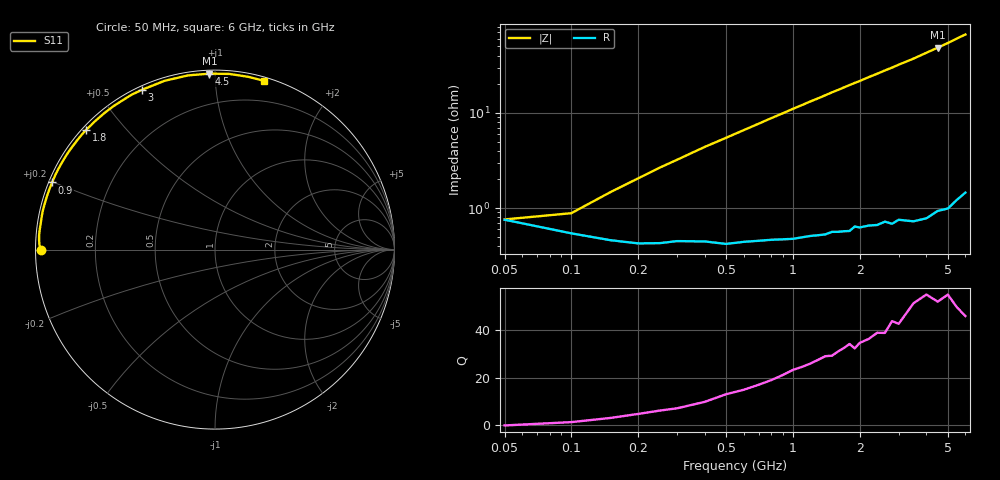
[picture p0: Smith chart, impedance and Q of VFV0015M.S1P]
! Infineon Technologies  Discrete & RF Semiconductors
! BBY 58-03
! Si Tuning Diode in SOD323
! VR =
! S-Parameters:  June  1999
# GHz  S  MA  R  50
!  f  S11
! GHz  MAG  ANG
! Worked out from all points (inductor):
!   34 points, 50 MHz to 6 GHz, reference 50 ohm
!   read as one part to ground: L = 1.6 nH near 150 MHz
!   highest Q = 54.8 at 4.5 GHz (marker M1), where L = 1.71 nH
!   S11 on the Smith chart (normalised r, x): 50 MHz: 0.02, -0.00; 900 MHz: 0.01, +0.20; 1.8 GHz: 0.01, +0.39; 3 GHz: 0.02, +0.64; 4.5 GHz: 0.02, +0.97; 6 GHz: 0.03, +1.33
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0.05  0.9702 -179.8
0.1  0.9785 178.4
0.15  0.9818 176.8
0.25  0.983 174.0
0.4  0.9824 170.0
0.5  0.9835 167.5
0.7  0.9824 162.5
0.8  0.9821 160.0
0.9  0.9821 157.6
1  0.982 155.1
1.2  0.9811 150.4
1.3  0.981 148.2
1.5  0.9799 143.6
1.6  0.9801 141.5
1.8  0.9803 137.2
1.9  0.9784 135.1
2  0.9791 133.2
2.2  0.9788 129.1
2.4  0.9792 125.4
2.6  0.9782 121.6
2.8  0.98 118.2
3  0.9789 114.6
3.5  0.9815 106.7
4  0.9821 98.8
4.5  0.9809 91.8
5  0.982 85.3
5.5  0.9803 79.1
6  0.9793 73.7
